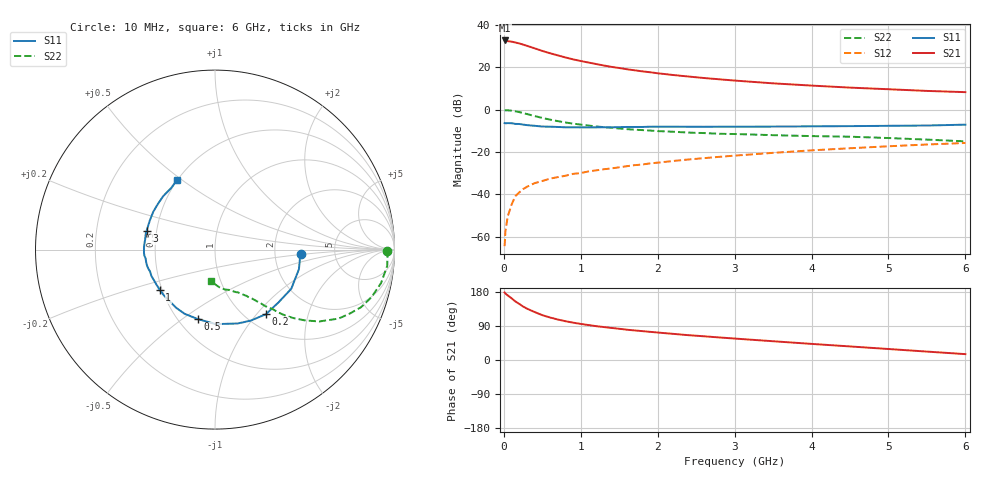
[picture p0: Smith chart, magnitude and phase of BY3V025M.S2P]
! SIEMENS Small Signal Semiconductors
! BFY420
! Si NPN RF SIEGET Grounded Emitter Transistor in MICRO-X
! VCE = 3 V  IC = 25 mA
! Common Emitter S-Parameters:  October  1996
# GHz  S  MA  R  50
!  f  S11  S21  S12  S22
! GHz  MAG  ANG  MAG  ANG  MAG  ANG  MAG  ANG
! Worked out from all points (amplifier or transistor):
!   36 points, 10 MHz to 6 GHz, reference 50 ohm
!   highest |S21| = 32.6 dB at 10 MHz (marker M1)
!   |S21| within 3 dB of that: start of sweep to 340.3 MHz
!   unconditionally stable (mu >= 1): 1.769 GHz to end of sweep
!   at 250 MHz: K = 0.33, MSG = 34.1 dB, |S12| = -37.5 dB
!   at 1.4 GHz: K = 0.94, MSG = 23.9 dB, |S12| = -27.7 dB
!   at 6 GHz: K = 1.06, MAG = 10.5 dB, |S12| = -15.7 dB
!   S11 on the Smith chart (normalised r, x): 10 MHz: 2.85, -0.17; 200 MHz: 1.23, -1.12; 500 MHz: 0.62, -0.57; 1 GHz: 0.49, -0.25; 3 GHz: 0.44, +0.11; 6 GHz: 0.50, +0.48
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0.01  0.4819 -2.8  42.84 178.2  0.0006 119.8  0.9583 -0.3
0.02  0.4757 -5.3  42.33 175.3  0.0013 87.7  0.9618 -1.5
0.05  0.4803 -13.2  41.2 170.6  0.003 86.8  0.9639 -5.4
0.1  0.4776 -27.2  40.21 163.0  0.0057 78.3  0.9438 -11.4
0.15  0.4601 -39.8  38.3 154.5  0.0091 74.4  0.9119 -16.8
0.2  0.4583 -51.7  36.47 148.1  0.0111 71.0  0.875 -21.5
0.25  0.4431 -63.2  34.24 141.2  0.0133 67.8  0.8291 -25.6
0.3  0.4307 -72.9  32.04 135.6  0.0151 67.6  0.7881 -29.2
0.4  0.4152 -89.5  27.95 126.6  0.0184 63.7  0.7053 -34.6
0.5  0.3987 -103.8  24.25 118.3  0.0207 61.6  0.6361 -38.3
0.6  0.3957 -115.4  21.41 112.2  0.0235 61.6  0.5806 -41.1
0.7  0.3896 -123.9  19.07 106.9  0.0255 60.9  0.536 -43.2
0.8  0.3824 -131.9  17.02 102.4  0.0275 60.3  0.4975 -44.8
1  0.381 -144.0  14.01 95.2  0.0319 60.5  0.4433 -47.0
1.1  0.3801 -149.6  12.9 92.2  0.0348 61.0  0.4211 -48.4
1.6  0.3895 -167.5  8.967 80.0  0.0463 60.6  0.3463 -52.6
2.2  0.3959 178.5  6.556 69.0  0.0614 59.0  0.3005 -57.4
3  0.3954 164.6  4.847 56.6  0.0821 54.8  0.2656 -63.4
3.5  0.3976 156.1  4.168 49.5  0.0955 51.6  0.2497 -67.4
4.5  0.4076 141.1  3.306 35.8  0.1226 43.5  0.2295 -75.9
5.5  0.4214 125.3  2.763 22.2  0.1502 34.4  0.1961 -88.7
6  0.442 118.7  2.583 15.5  0.1633 29.6  0.1783 -97.4
